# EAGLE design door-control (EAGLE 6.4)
REV: A; TITLE: RPi + CC2520
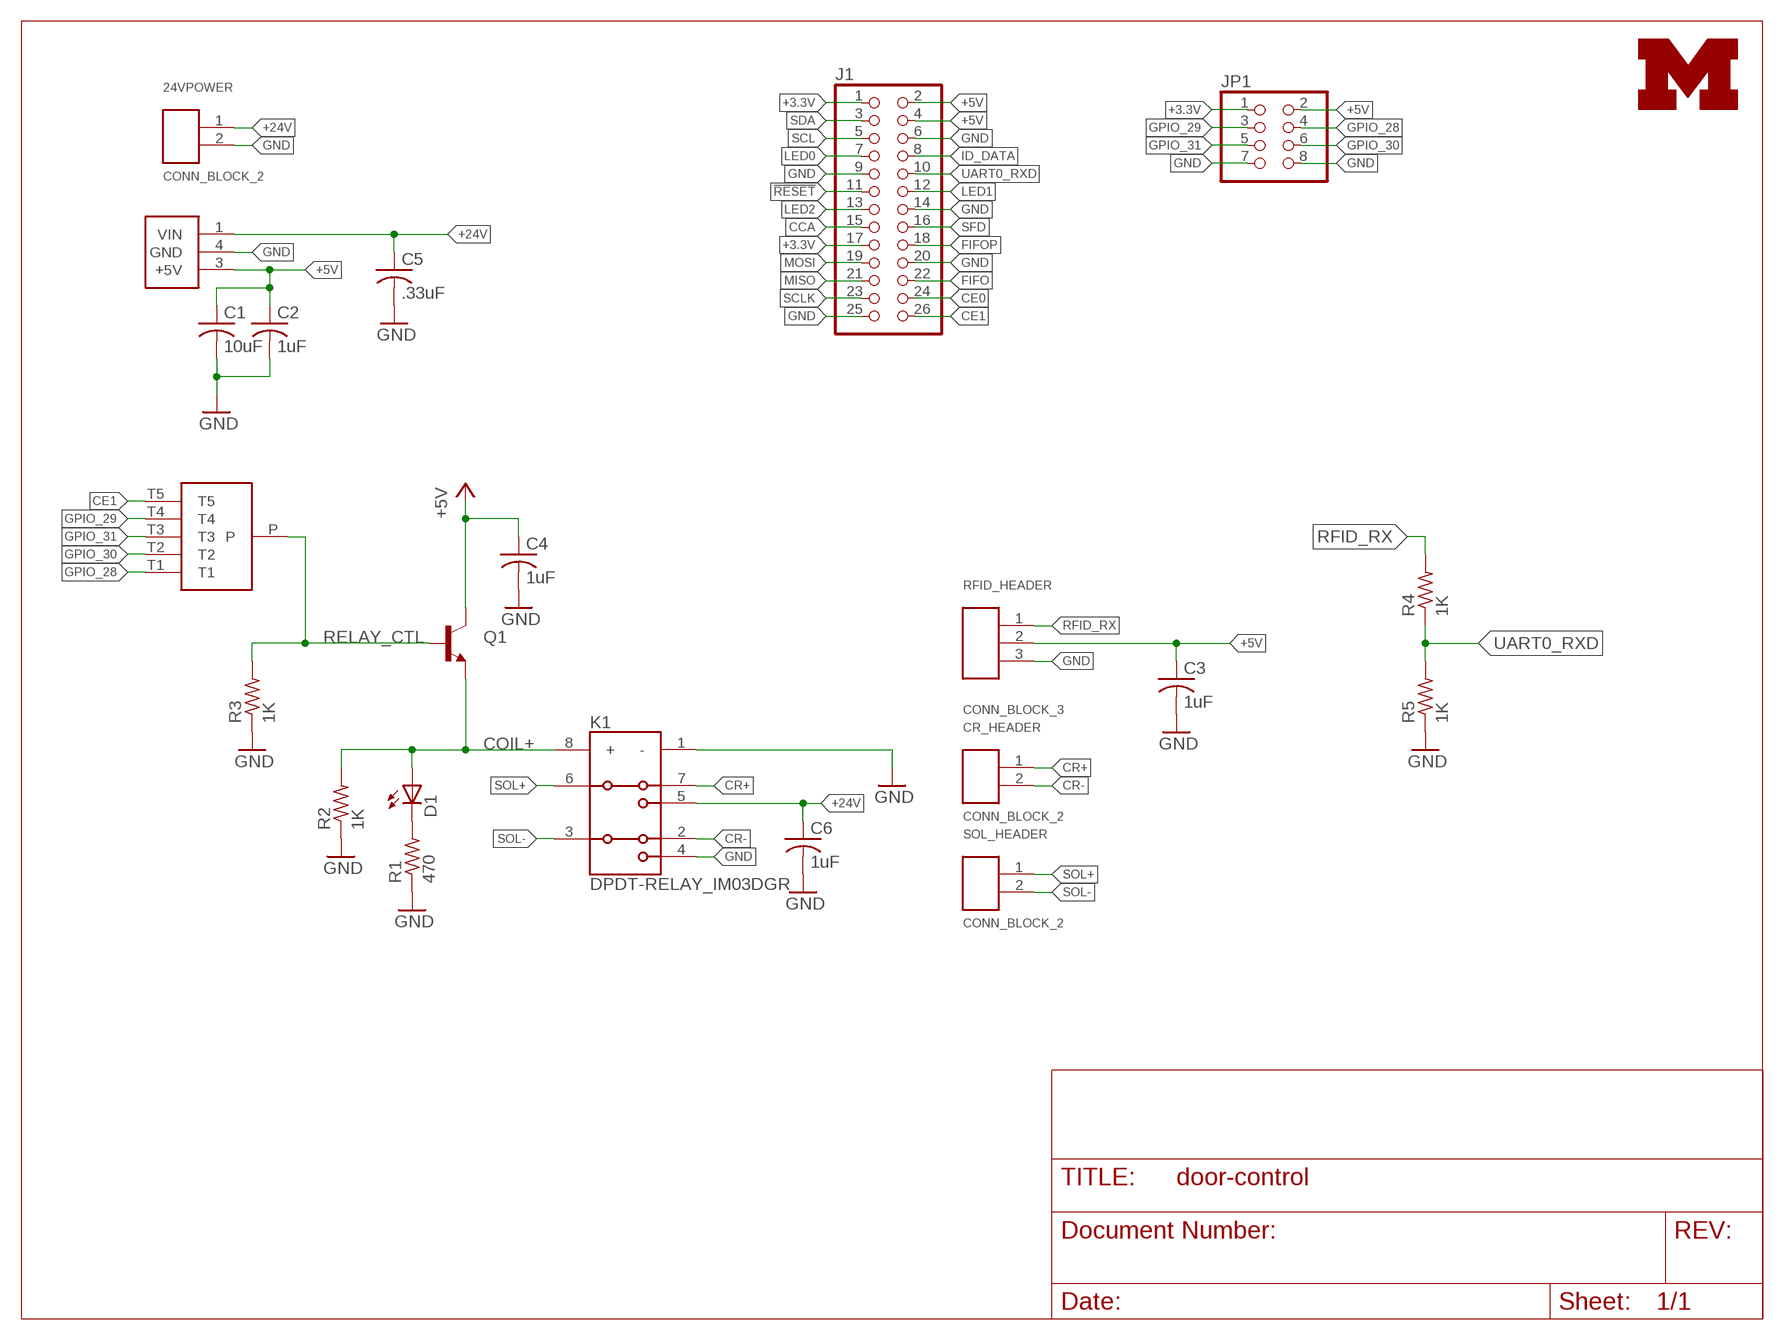
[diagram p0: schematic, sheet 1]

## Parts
24VPOWER  CONN_BLOCK_2  [CONN_BLOCK_2]
C1  10uF  C-USC0603  [C0603]
C2  1uF  C-USC0603  [C0603]
C3  1uF  C-USC0603  [C0603]
C4  1uF  C-USC0603  [C0603]
C5  .33uF  C-USC0603  [C0603]
C6  1uF  C-USC0603  [C0603]
CR_HEADER  CONN_BLOCK_2  [CONN_BLOCK_2]
D1  LED0603  [LED-0603]
J1  PINHD-2X13  [2X13]
JP1  PINHD-2X4  [2X04]
K1  DPDT-RELAY_IM03DGR  [TE-DPDT-RELAY]
Q1  TRANSISTOR_NPNSOT23  [SOT23]
R1  470  R-US_R0402  [R0402]
R2  1K  R-US_R0402  [R0402]
R3  1K  R-US_R0402  [R0402]
R4  1K  R-US_R0402  [R0402]
R5  1K  R-US_R0402  [R0402]
RFID_HEADER  CONN_BLOCK_3  [CONN_BLOCK_3]
S1  SP5T_RESISTORS  [SP5T_0603_RESISTORS]
SOL_HEADER  CONN_BLOCK_2  [CONN_BLOCK_2]
U$1  UMICH_SOLID_SMALL  [UMICH_SOLID_75MIL]
VR1  LDO_TO_5V  [TO-252-3,SO-63]

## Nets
!RESET: J1.11
+3.3V: J1.1 J1.17 JP1.1
+5V: C1.1 C2.1 C3.1 C4.1 J1.2 J1.4 JP1.2 Q1.3(C) RFID_HEADER.2 VR1.3(+5V)
+24V: 24VPOWER.1 C5.1 C6.1 K1.5(Z1) VR1.1(VIN)
CCA: J1.15
CE0: J1.24
CE1: J1.26 S1.T5
COIL+: D1.A K1.8(+) Q1.2(E) R2.2
CR+: CR_HEADER.1 K1.7(Y1)
CR-: CR_HEADER.2 K1.2(Y2)
FIFO: J1.22
FIFOP: J1.18
GND: 24VPOWER.2 C1.2 C2.2 C3.2 C4.2 C5.2 C6.2 J1.6 J1.9 J1.14 J1.20 J1.25 JP1.7 JP1.8 K1.1(-) K1.4(Z2) R1.1 R2.1 R3.1 R5.1 RFID_HEADER.3 VR1.4(GND)
GPIO_28: JP1.4 S1.T1
GPIO_29: JP1.3 S1.T4
GPIO_30: JP1.6 S1.T2
GPIO_31: JP1.5 S1.T3
ID_DATA: J1.8
LED0: J1.7
LED1: J1.12
LED2: J1.13
MISO: J1.21
MOSI: J1.19
N$1: D1.C R1.2
RELAY_CTL: Q1.1(B) R3.2 S1.P
RFID_RX: R4.2 RFID_HEADER.1
SCL: J1.5
SCLK: J1.23
SDA: J1.3
SFD: J1.16
SOL+: K1.6(A1) SOL_HEADER.1
SOL-: K1.3(A2) SOL_HEADER.2
UART0_RXD: J1.10 R4.1 R5.2

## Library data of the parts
24VPOWER CR_HEADER SOL_HEADER = door-control:CONN_BLOCK_2: 2x 0.100 in screw terminal block; DIGIKEY: 277-1273-ND
C1-C6 = resistor:C-US: CAPACITOR, American symbol
D1 = SparkFun-LED:LED: LEDs; DIGIKEY: 160-1834-1-ND
J1 = pinhead:PINHD-2X13: PIN HEADER; DIGIKEY: SAM1204-13-ND
JP1 = pinhead:PINHD-2X4: PIN HEADER
K1 = door-control:DPDT-RELAY_IM03DGR; DIGIKEY: PB1172CT-ND
Q1 = door-control:TRANSISTOR_NPN: Transistor NPN BJT configuration in SOT23 package. MMBT2222 is the common NPN we use. Double check BCE configuration again layout.
R1-R5 = rcl:R-US_: RESISTOR, American symbol; DIGIKEY: RHM470JCT-ND
RFID_HEADER = door-control:CONN_BLOCK_3: 3x 0.100 in screw terminal block; DIGIKEY: 277-1274-ND
S1 = door-control:SP5T_RESISTORS
U$1 = logos:UMICH_SOLID
VR1 = door-control:LDO_TO_5V; DIGIKEY: MC7805CDTRKGOSCT-ND

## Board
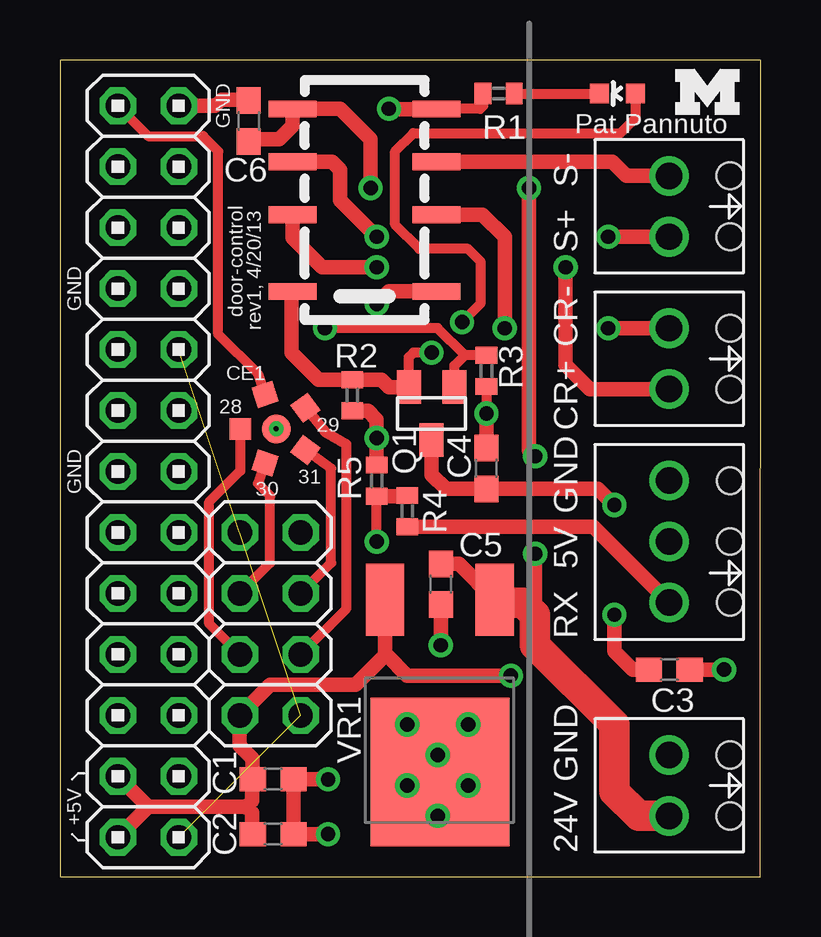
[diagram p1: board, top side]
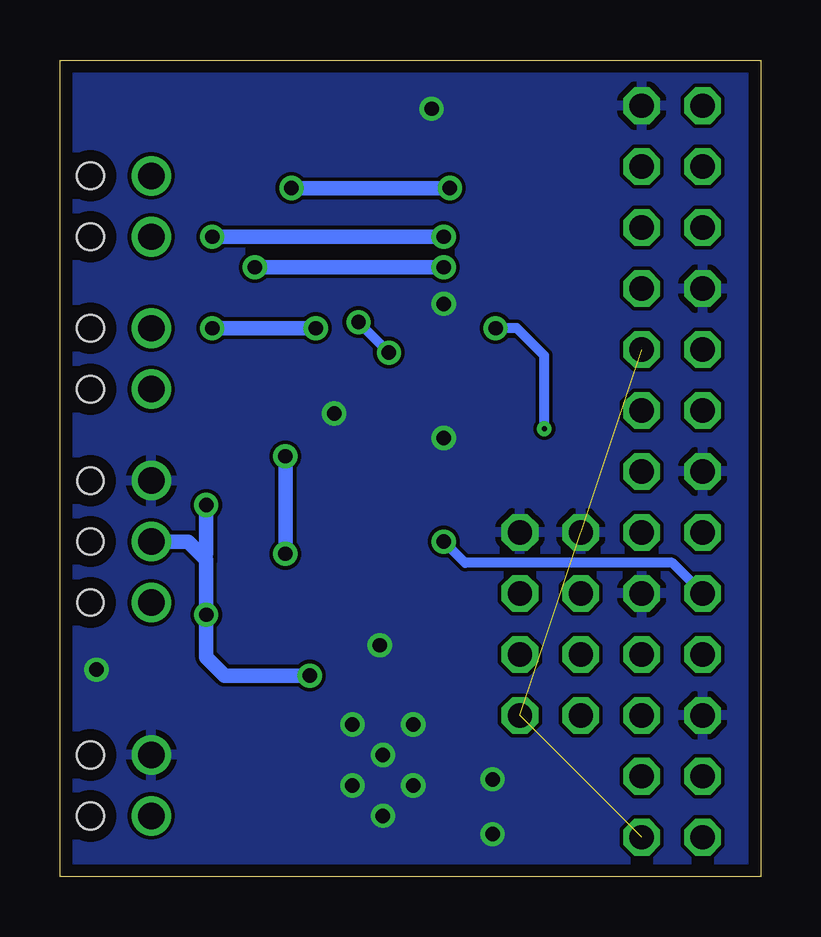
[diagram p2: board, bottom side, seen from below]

Size 29.21 x 34.04 mm. Coordinates in mm from the lower left corner, seen from the top.
Outline: 0,0 29.19,0 29.21,34.04 0,34.04 0,0
Copper layers (1*16): Top 0.0178mm / dielectric 59mil / Bottom 0.0178mm
Design rules "sunstone-2lyr_v1.0.0.3 *": minimum track width 6mil, minimum drill 14mil, track to track 6mil, track to pad 6mil, pad to pad 6mil, via to via 6mil, smd to smd 6mil, copper to edge 20mil, drill to drill 16mil, minimum pad ring 8mil, minimum via ring 8mil, stop-mask expansion 3mil, vias tented up to drill 24mil, thermal gap 10mil

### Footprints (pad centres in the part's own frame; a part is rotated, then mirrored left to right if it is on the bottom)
CONN_BLOCK_2 = drill 1.1: 1 -1.27,0; 2 1.27,0 | hole 1.12: -1.27,-2.54; 1.27,-2.54
C0603 = smd 1.1 x 1: 1 -0.85,0; 2 0.85,0
LED-0603 = smd 0.8 x 0.8: A 0,-0.75; C 0,0.75
2X13 = drill 1.016 octagon: 1 -15.24,-1.27; 2 -15.24,1.27; 3 -12.7,-1.27; 4 -12.7,1.27; 5 -10.16,-1.27; 6 -10.16,1.27; 7 -7.62,-1.27; 8 -7.62,1.27; 9 -5.08,-1.27; 10 -5.08,1.27; 11 -2.54,-1.27; 12 -2.54,1.27; 13 0,-1.27; 14 0,1.27; 15 2.54,-1.27; 16 2.54,1.27; 17 5.08,-1.27; 18 5.08,1.27; 19 7.62,-1.27; 20 7.62,1.27; 21 10.16,-1.27; 22 10.16,1.27; 23 12.7,-1.27; 24 12.7,1.27; 25 15.24,-1.27; 26 15.24,1.27
2X04 = drill 1.016 octagon: 1 -3.81,-1.27; 2 -3.81,1.27; 3 -1.27,-1.27; 4 -1.27,1.27; 5 1.27,-1.27; 6 1.27,1.27; 7 3.81,-1.27; 8 3.81,1.27
TE-DPDT-RELAY = smd 0.7 x 2: 1 -3.8,-3; 2 -0.6,-3; 3 1.6,-3; 4 3.8,-3; 5 3.8,3; 6 1.6,3; 7 -0.6,3; 8 -3.8,3
SOT23 = smd 1 x 1.4: 1 -0.95,-1.1; 2 0.95,-1.1; 3 0,1.1
R0402 = smd 0.7 x 0.9: 1 -0.65,0; 2 0.65,0
CONN_BLOCK_3 = drill 1.1: 1 -2.54,0; 2 0,0; 3 2.54,0 | hole 1.1: -2.54,-2.54; 0,-2.54; 2.54,-2.54
SP5T_0603_RESISTORS = smd 1.2 x 1.2: P 0,0 | smd 0.9 x 0.9: T1 1.5,0 | smd 0.9 x 0.9 rotated 72: T2 0.464,1.427 | smd 0.9 x 0.9 rotated 144: T3 -1.214,0.882 | smd 0.9 x 0.9 rotated 216: T4 -1.214,-0.882 | smd 0.9 x 0.9 rotated 288: T5 0.464,-1.427
TO-252-3,SO-63 = smd 3 x 1.6: 1 10.28,0.8; 3 10.28,5.37 | smd 6.2 x 5.8: 4 3.1,3.085

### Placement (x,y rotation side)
24VPOWER  25.4,3.81 90 top
C1  8.89,4.06 0 top
C2  8.89,1.78 0 top
C3  25.4,8.64 0 top
C4  17.78,17.02 90 top
C5  15.88,12.19 270 top
C6  7.87,31.5 90 top
CR_HEADER  25.4,21.59 90 top
D1  23.24,32.64 90 top
J1  3.68,16.89 90 top
JP1  8.76,10.54 90 top
K1  12.7,28.19 90 top
Q1  15.49,19.3 180 top
R1  18.29,32.64 0 top
R2  12.19,20.07 90 top
R3  17.78,21.08 90 top
R4  14.48,15.24 270 top
R5  13.21,16.51 270 top
RFID_HEADER  25.4,13.97 90 top
S1  9.02,18.67 180 top
SOL_HEADER  25.4,27.94 90 top
U$1  25.65,31.75 0 top
VR1  18.92,1.27 90 top

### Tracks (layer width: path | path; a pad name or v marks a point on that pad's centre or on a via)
+3.3V  (2 unrouted)
+5V  (via drill 0.6)
  Top 0.61: C3.1 23.88,8.64 23.11,9.4 v23.11,10.92 | VR1.3 13.55,9.23 | 13.55,9.23 12.32,8 8.76,8 JP1.2 7.49,5.46 8.04,4.91 C1.1 | J1.2 3.68,2.92 | 3.68,2.92 J1.4 | 3.68,2.92 7.75,2.92 | 7.75,2.92 8,2.67 8,1.82 C2.1 | 7.75,2.92 8,3.17 8,4.03 C1.1 | 8.13,3.98 C1.1 | v23.11,15.49 22.44,16.17 C4.1 16.09,16.17 15.49,16.76 Q1.3 | 13.55,9.23 13.62,9.23 14.48,8.38 v18.8,8.38
  Bottom 0.61: 23.24,13.34 23.11,13.21 v23.11,10.92 23.11,9.14 22.35,8.38 v18.8,8.38 | 23.24,13.34 23.88,13.97 RFID_HEADER.2 | v23.11,15.49 23.11,13.46 23.24,13.34
+24V  (via drill 0.6)
  Top 0.61: v12.95,28.7 12.95,30.73 11.68,32 9.71,32 K1.5 9.7,31.29 9.14,30.73 8.04,30.73 C6.1 | v19.56,28.7 19.56,17.78 v19.81,17.53 | v19.81,13.46 19.81,10.92 | C5.1 16.63,13.04 VR1.1
  Top 1.27: 24VPOWER.1 24.13,2.54 23.11,3.56 23.11,6.35 19.81,9.65 19.81,10.92 19.3,11.43 18.24,11.43 VR1.1
  Bottom 0.61: v19.56,28.7 v12.95,28.7 | v19.81,17.53 v19.81,13.46
CE1
  Top 0.406: J1.26 3.68,30.86 5.97,30.86 6.6,30.23 6.6,22.61 8.26,20.95 S1.T5
COIL+  (via drill 0.6)
  Top 0.406: D1.A 23.99,31.61 23.37,30.99 14.73,30.99 13.97,30.23 13.97,27.18 14.99,26.16 17.02,26.16 17.53,25.65 17.53,23.88 v16.76,23.11 | 9.65,24.35 K1.8 | 13.72,20.4 13.63,20.4 13.46,20.57 | v15.49,21.84 14.73,21.84 14.54,21.66 Q1.2
  Top 0.61: 9.65,24.35 9.65,21.84 10.78,20.72 R2.2 13.4,20.72 13.72,20.4 Q1.2
  Bottom 0.406: v16.76,23.11 v15.49,21.84
CR+  (via drill 0.6)
  Top 0.61: K1.7 9.7,26.62 10.92,25.4 v13.21,25.4 | v21.08,25.4 21.08,21.34 22.1,20.32 CR_HEADER.1
  Bottom 0.61: v13.21,25.4 v21.08,25.4
CR-  (via drill 0.6)
  Top 0.61: K1.2 17.62,27.59 18.54,26.67 v18.54,22.86 | v22.86,22.86 CR_HEADER.2
  Bottom 0.61: v18.54,22.86 v22.86,22.86
GND  (via drill 0.6)
  Top 0.406: VR1.4 15.84,4.99 v15.75,5.08 | R1.1 17.64,32.12 17.53,32 15.71,32 K1.4 | R3.1 v17.78,19.3
  Top 0.61: C3.2 v27.69,8.64 | K1.4 v13.73,31.99 v13.72,32 | K1.1 13.73,24.39 v13.21,23.88 | v11.18,4.06 C1.2 9.74,1.94 9.91,1.78 | v11.18,1.78 9.91,1.78 | 9.91,1.78 C2.2 | R5.1 v13.21,18.29 13.21,19.05 12.84,19.42 R2.1 | C5.2 v15.88,9.65 | C4.2 v17.78,19.3 | J1.25 6.48,32.13 6.73,32.38 7.83,32.38 C6.2
  other vias: 14.48,6.35 17.02,6.35 14.48,3.81 17.02,3.81 15.75,2.54
  pour Bottom: 0,0 0,34.04 29.21,34.04 29.21,0
GPIO_28
  Top 0.406: JP1.4 6.22,10.54 6.22,15.62 7.52,16.91 S1.T1
GPIO_29
  Top 0.406: JP1.3 11.94,11.18 11.94,18.03 11.05,18.54 S1.T4
GPIO_30
  Top 0.406: JP1.6 8.76,13.08 8.76,15.88 8.26,16.38 S1.T2
GPIO_31
  Top 0.406: JP1.5 11.3,13.08 11.3,17.02 S1.T3
N$1
  Top 0.406: R1.2 D1.C
RELAY_CTL  (via drill 0.2, 0.6)
  Top 0.406: 16.88,21.73 15.75,22.86 v11.05,22.86 | R3.2 16.88,21.73 | Q1.1 16.44,21.3 16.88,21.73
  Bottom 0.406: S1.P 9.02,21.72 10.16,22.86 v11.05,22.86
  other vias: 9.02,18.67
RFID_RX
  Top 0.61: R4.2 22.24,14.59 RFID_HEADER.1
SOL+  (via drill 0.6)
  Top 0.61: K1.6 11.35,29.79 11.68,29.46 11.68,28.19 v13.21,26.67 | v22.86,26.67 SOL_HEADER.1
  Bottom 0.61: v13.21,26.67 v22.86,26.67
SOL-
  Top 0.61: K1.3 23.04,29.79 23.62,29.21 SOL_HEADER.2
UART0_RXD  (via drill 0.6)
  Top 0.406: v13.21,13.97 R5.2 | 14.45,15.86 R4.1
  Top 0.61: R5.2 14.45,15.86
  Bottom 0.406: J1.10 3.68,13.08 12.32,13.08 v13.21,13.97

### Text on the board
tPlace: GND | Pat Pannuto | S- | S+ | door-control | GND | rev1, 4/20/13 | CR- | CE1 | CR+ | 28 | 29 | GND | GND | 30 | 31 | 5V | RX | GND | +5V | 24V
tDocu: CC2520 Edge

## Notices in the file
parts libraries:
SparkFun-LED: Licensing: CC v3.0 Share-Alike You are welcome to use this library for commercial purposes.
